FUNCTION_BLOCK SDOread
	VAR_INPUT
   ADSNetID:STRING(23); (* The AMSNetID addresses the EL6751. Can be empty if only one local single channel card is present*)

   PortNr:WORD;         (* This Port No. addresses the CANopen Node (see System Manager) *)

   CO_Index:DWORD;      (* This is the Index of the CANopen Object Dictionary Entry*)

   CO_SubIndex:DWORD;   (* This is the Sub-Index of the CANopen Object Dictionary Entry*)

   DataLength:DWORD;    (* This is the Length of the CANopen Object Dictionary Entry*)

   StartReading:BOOL;   (* only reset to FALSE after ReadDataAvailable=TRUE*)

END_VAR

VAR_OUTPUT
   ReadData:ARRAY[0..255] OF BYTE;
   ReadDataAvailable:BOOL;
   Error:DWORD;
END_VAR

VAR
   state:BYTE := 0;
   ADSREAD:ADSREAD;
END_VAR

CASE state OF
0:
	IF StartReading THEN
	   ReadDataAvailable := FALSE;
	   Error := 0;
	   ADSRead(
		   NETID:= ADSNetID,
		   PORT:= PortNr,
		   IDXGRP:= CO_Index,
		   IDXOFFS:= CO_SubIndex,
		   LEN:= DataLength,
		   DESTADDR:= ADR(ReadData),
		   READ:= TRUE,
		   TMOUT := T#1s
		   );
	   IF ADSRead.err THEN
		   state := 2;
		   ReadDataAvailable := TRUE;
		   Error := ADSRead.ErrId;
	   ELSE
		   state := 1;
	   END_IF
	ELSE
	   ADSRead(
		   NETID:= ADSNetID,
		   PORT:= PortNr,
		   IDXGRP:= CO_Index,
		   IDXOFFS:= CO_SubIndex,
		   LEN:= DataLength,
		   DESTADDR:= ADR(ReadData),
		   READ:= FALSE,
		   TMOUT := T#1s
	   );
	END_IF
1:
	ADSRead(READ:= FALSE);
	IF ADSRead.err THEN
	   state := 2;
	   ReadDataAvailable := TRUE;
	   Error := ADSRead.ErrId;
	ELSE
	   IF NOT ADSRead.busy THEN
		   state := 2;
		   ReadDataAvailable := TRUE;
	   END_IF
	END_IF
2:
	ADSRead(READ:= FALSE);
	state := 0;
END_CASE

END_FUNCTION_BLOCK
